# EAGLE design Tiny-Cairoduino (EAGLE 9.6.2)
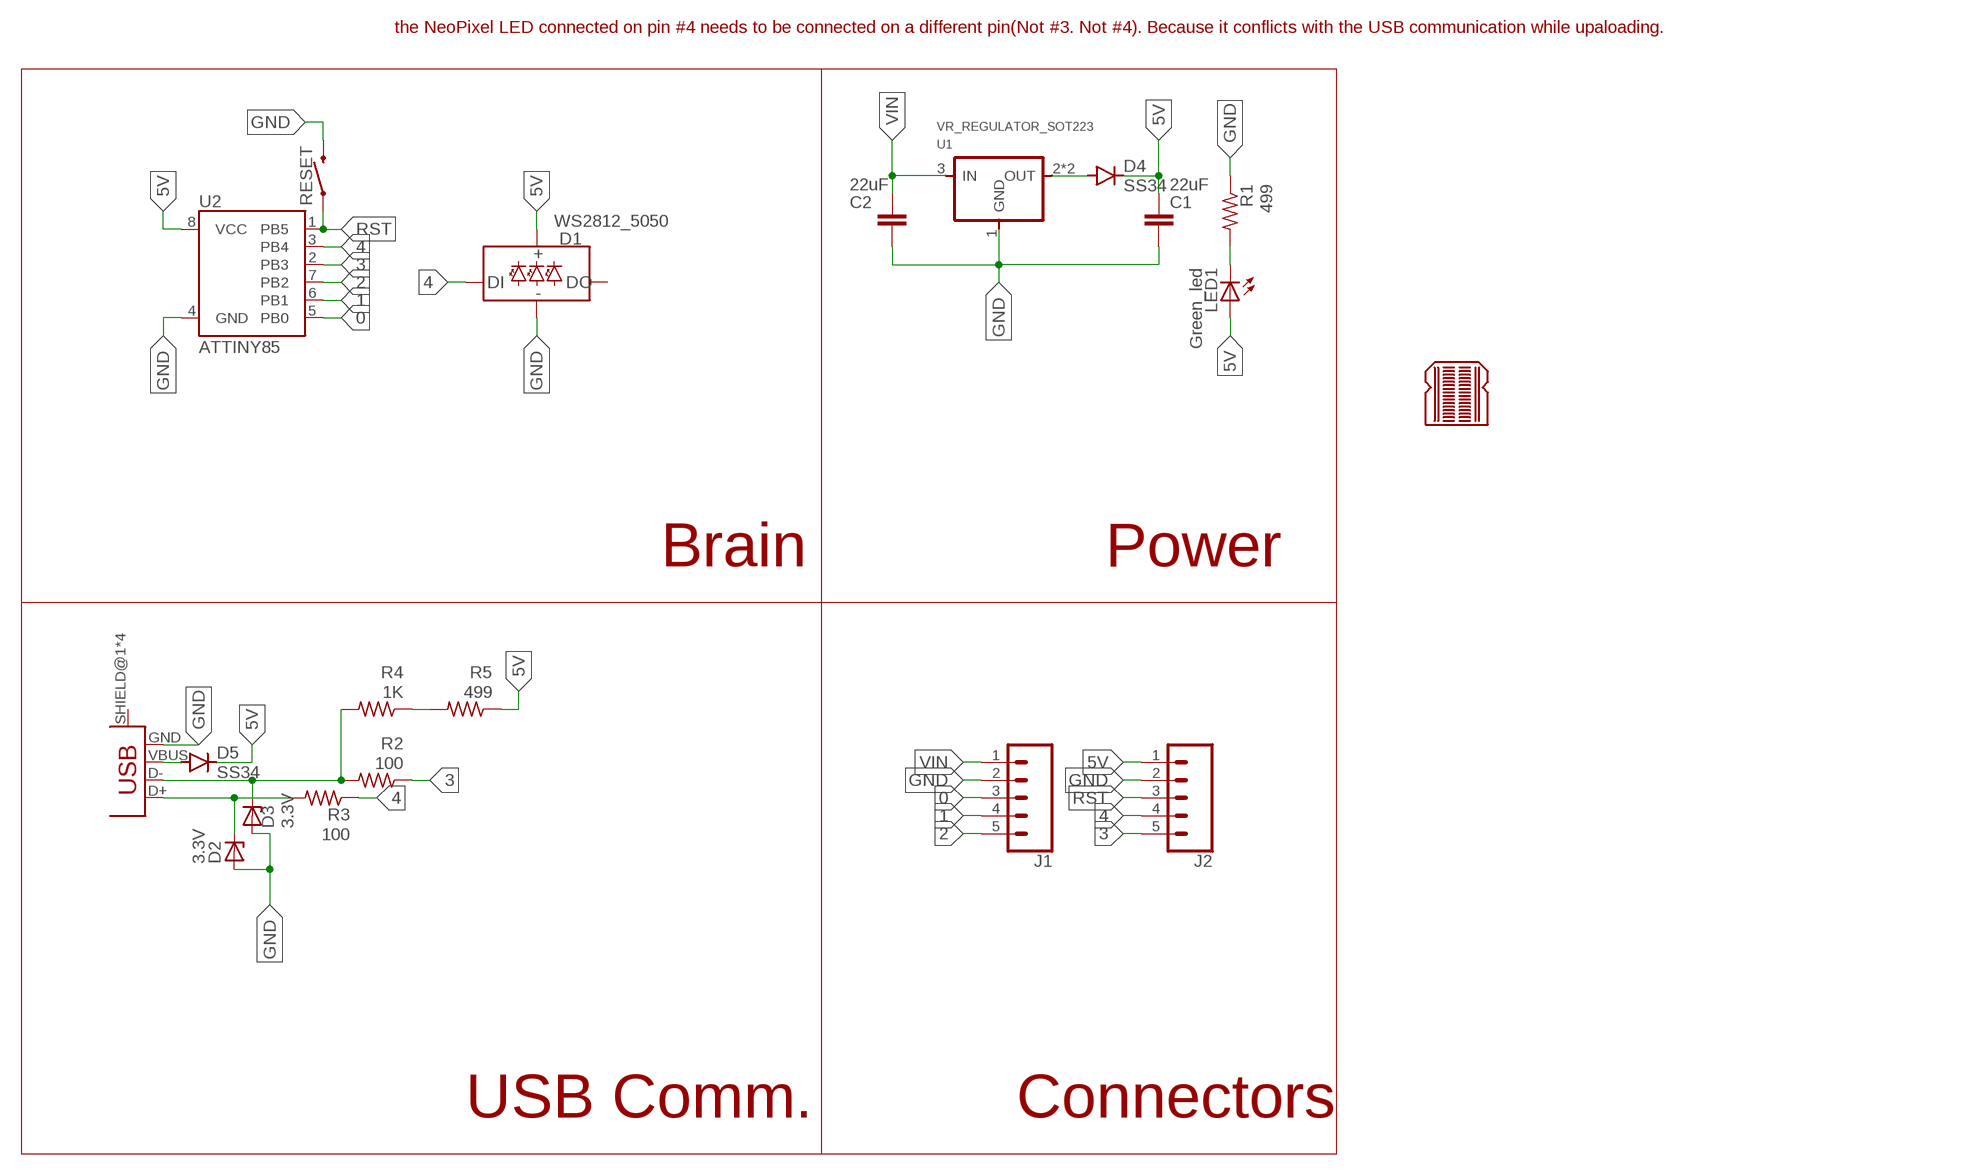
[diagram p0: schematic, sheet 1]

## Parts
C1  22uF  22UF-0805-16V-20%  [0805]
C2  22uF  22UF-0805-16V-20%  [0805]
D1  WS2812_5050  [WS2812-5X5-4PIN]
D2  3.3V  DIODE_ZENERSOD123  [SOD123]
D3  3.3V  DIODE_ZENERSOD123  [SOD123]
D4  SS34  DIODE-DO-214AC  [DO-214AC]
D5  SS34  DIODE-DO-214AC  [DO-214AC]
J1  CONN_05  [1X05]
J2  CONN_05  [1X05]
LED1  Green_led  LEDCHIP-LED0805  [CHIP-LED0805]
LOGO1  BREADBOARD_PATTERN  [BREADBOARD_SPACING]
R1  499  R1206FAB  [R1206FAB]
R2  100  R1206FAB  [R1206FAB]
R3  100  R1206FAB  [R1206FAB]
R4  1K  R1206FAB  [R1206FAB]
R5  499  R1206FAB  [R1206FAB]
RESET  MOMENTARY-SWITCH-SPST-SMD-6.0X3.5MM  [TACTILE_SWITCH_SMD_6.0X3.5MM]
U1  VR_REGULATOR_SOT223  [SOT223]
U2  ATTINY85  [ATTINY85]
U$2  CONN_USB_MINIB  [USB_MINIB]

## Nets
0: J1.3 U2.5(PB0)
1: J1.4 U2.6(PB1)
2: J1.5 U2.7(PB2)
3: J2.5 R2.1 U2.2(PB3)
4: D1.DI J2.4 R3.1 U2.3(PB4)
5V: C1.1 D1.VCC D4.C D5.C J2.1 LED1.A R5.1 U2.8(VCC)
GND: C1.2 C2.2 D1.GND D2.ANODE D3.ANODE J1.2 J2.2 R1.1 RESET.2 U1.1(GND) U2.4(GND) U$2.GND
N$1: LED1.C R1.2
N$2: D5.A U$2.VBUS
N$3: R4.1 R5.2
N$4: D3.CATHODE R2.2 R4.2 U$2.D-
N$5: D2.CATHODE R3.2 U$2.D+
N$6: D4.A U1.2(OUT) U1.4(OUT)
RST: J2.3 RESET.1 U2.1(PB5)
VIN: C2.1 J1.1 U1.3(IN)
Unconnected: D1.DO U$2.SHIELD@1(SHIELD) U$2.SHIELD@2(SHIELD) U$2.SHIELD@3(SHIELD) U$2.SHIELD@4(SHIELD)

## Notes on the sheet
- the NeoPixel LED connected on pin #4 needs to be connected on a different pin(Not #3. Not #4). Because it conflicts with the USB communication while upaloading.
- Brain | Power
- USB Comm. | Connectors

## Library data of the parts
C1 C2 = SparkFun-Capacitors:22UF: 22µF ceramic capacitors; PROD_ID: CAP-14260
D1 = SparkFun-LED:WS2812: Addressable RGB LED - 1 Wire Common names: WS2812, SK6812, Neopixel, APA-106, etc. SMD LED with built-in controller IC. Color: Red/Green/Blue SparkFun Products: LED-SMD RGB (WS2812) LED - RGB Addressable, PTH, 5mm Diffused (5 Pack) LED - RGB Addressable, PTH, 5mm Clear (5 Pack) Blynk Board -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; PROD_ID: DIO-12503
D2 D3 = fab:DIODE_ZENER: zener diode
D4 D5 = diode:DIODE-: DIODE
J1 J2 = SparkFun-Connectors:CONN_05: Multi connection point. Often used as Generic Header-pin footprint for 0.1 inch spaced/style header connections On any of the 0.1 inch spaced packages, you can populate with these: Break Away Headers - Straight (PRT-00116) Break Away Male Headers - Right Angle (PRT-00553) Female Headers (PRT-00115)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
LED1 = adafruit:LED: LED
LOGO1 = SparkFun-Aesthetics:BREADBOARD_PATTERN: Breadboard-Spacing Reference
R1-R5 = fab:R: Resistor (US Symbol)
RESET = SparkFun-Switches:MOMENTARY-SWITCH-SPST: Momentary Switch (Pushbutton) - SPST; PROD_ID: SWCH-14278; SF_SKU: COM-08229
U1 = fab:VR_REGULATOR_SOT223
U2 = SparkFun-IC-Microcontroller:ATTINY85; PROD_ID: IC-09092
U$2 = fab:CONN_USB_MINIB

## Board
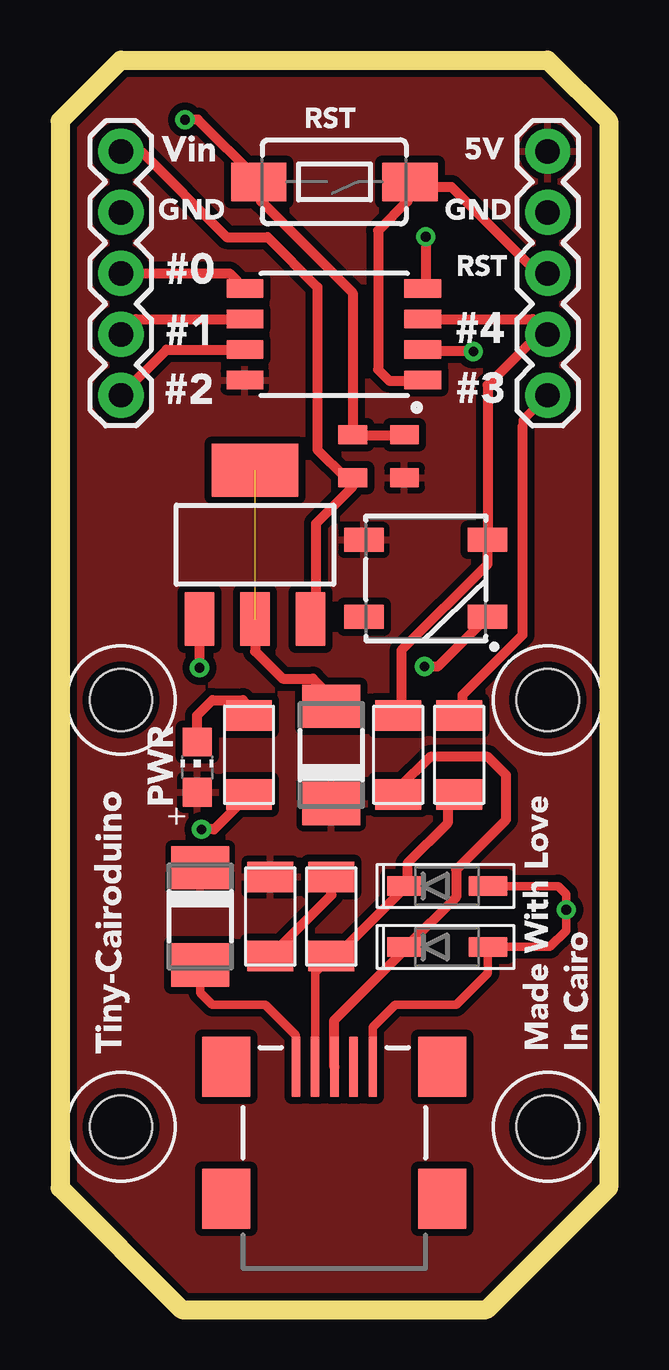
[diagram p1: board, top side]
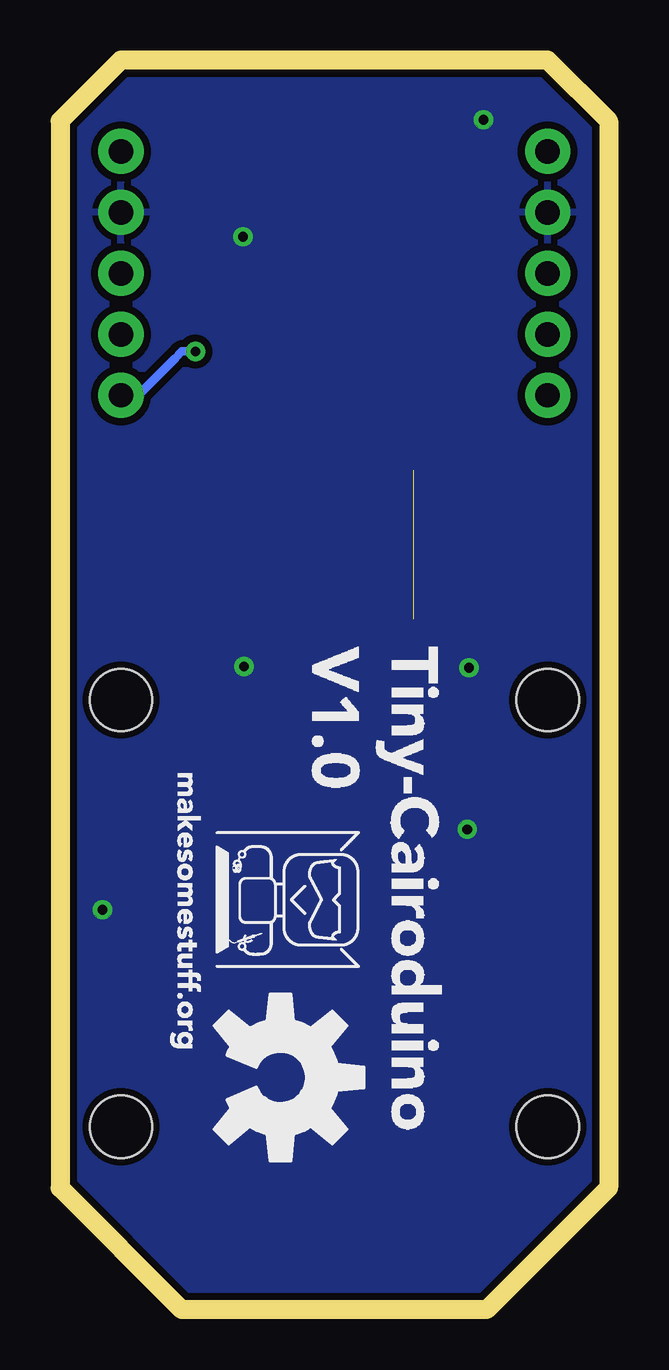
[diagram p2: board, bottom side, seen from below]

Size 22.86 x 52.07 mm. Coordinates in mm from the lower left corner, seen from the top.
Outline: 0,49.53 2.54,52.07 20.32,52.07 22.86,49.53 22.86,5.08 17.78,0 5.08,0 0,5.08 0,49.53
Copper layers (1*16): Top 0.035mm / dielectric 1.5mm / Bottom 0.035mm
Design rules "default *": minimum track width 0.3mm, minimum drill 0.3mm, track to track 10mil, track to pad 10mil, pad to pad 10mil, via to via 10mil, smd to smd 10mil, copper to edge 10mil, drill to drill 10mil, minimum pad ring 10mil, minimum via ring 8mil, stop-mask expansion 4mil, vias tented up to drill 0mil, thermal gap 10mil
Holes 2.6 mm at 20.32,7.62 2.54,7.62 20.32,25.4 2.54,25.4

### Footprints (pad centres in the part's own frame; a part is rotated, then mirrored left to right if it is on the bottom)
0805 = smd 0.8 x 1.2: 1 -0.9,0; 2 0.9,0
WS2812-5X5-4PIN = smd 1.651 x 1: DI 2.577,1.6; DO -2.577,-1.6; GND 2.577,-1.6; VCC -2.577,1.6
SOD123 = smd 1.6 x 0.8: ANODE 1.7,0; CATHODE -1.7,0
DO-214AC = smd 1.8 x 2.4: A 2.025,0; C -2.025,0
1X05 = drill 1.016 pad 1.88: 1 0,0; 2 2.54,0; 3 5.08,0; 4 7.62,0; 5 10.16,0
CHIP-LED0805 = smd 1.2 x 1.2: A 0,-1.05; C 0,1.05
R1206FAB = smd 1.27 x 1.905: 1 -1.651,0; 2 1.651,0
TACTILE_SWITCH_SMD_6.0X3.5MM = smd 2.3 x 1.6: 1 -3.15,0; 2 3.15,0
SOT223 = smd 1.219 x 2.235: 1 -2.311,-3.099; 2 0,-3.099; 3 2.311,-3.099 | smd 3.6 x 2.2: 4 0,3.099
ATTINY85 = smd 1.524 x 0.762: 1 -3.683,1.905; 2 -3.683,0.635; 3 -3.683,-0.635; 4 -3.683,-1.905; 5 3.727,-1.905; 6 3.727,-0.635; 7 3.727,0.635; 8 3.727,1.905
USB_MINIB = smd 2.5 x 0.35: D+ 3.77,0; D- 3.77,0.8; GND 3.77,-1.6; ID 3.77,-0.8; VBUS 3.77,1.6 | smd 2.5 x 2: SHIELD@1 -1.73,-4.5; SHIELD@2 -1.73,4.5; SHIELD@3 3.77,4.5; SHIELD@4 3.77,-4.5

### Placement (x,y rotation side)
C1  14.35,35.56 90 top
C2  12.19,35.56 90 top
D1  15.24,30.48 0 top
D2  16.13,15.11 0 top
D3  16.13,17.65 0 top
D4  11.3,23.11 90 top
D5  5.84,16.38 270 top
J1  2.54,48.26 270 top
J2  20.32,48.26 270 top
LED1  5.71,22.61 0 top
LOGO1  not placed on the board
R1  7.87,23.11 90 top
R2  16.64,23.11 270 top
R3  14.1,23.11 270 top
R4  11.3,16.38 270 top
R5  8.76,16.38 270 top
RESET  11.43,46.99 180 top
U1  8.13,31.88 0 top
U2  11.43,40.64 180 top
U$1  [OSHW-LOGO-L]  13.68,9.68 270 bottom
U$2  11.43,6.35 90 top

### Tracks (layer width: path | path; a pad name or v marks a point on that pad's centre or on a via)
0
  Top 0.406: J1.3 7.07,43.18 U2.5
1
  Top 0.406: J1.4 3.17,41.27 U2.6
2
  Top 0.406: J1.5 4.45,40.01 U2.7
3  (via drill 0.4)
  Top 0.35: 19.28,36.8 19.28,37.06 J2.5
  Top 0.406: v17.22,39.93 15.24,39.93 U2.2 | R2.1 16.76,24.84 16.76,25.6 19.28,28.12 19.28,36.8
  Bottom 0.35: J2.5 19.61,38.1 18.06,39.65 17.78,39.93 v17.22,39.93
4
  Top 0.406: R3.1 14.22,24.89 14.22,27.47 17.82,31.06 D1.DI 17.82,38.52 19.94,40.64 J2.4 19.68,41.27 U2.3
5V
  pour Top (isolate 0.3): 5.08,0 0,5.08 0,49.53 2.54,52.07 20.32,52.07 22.86,49.53 22.86,5.08 17.78,0
GND  (via drill 0.4)
  Top 0.35: U$2.GND 13.03,11.76 13.97,12.7 16.51,12.7 17.83,14.02 D2.ANODE 20.41,15.11 21.09,15.8 v21.09,16.66 21.09,17.31 20.75,17.65 D3.ANODE
  Top 0.406: 17.83,17.53 D3.ANODE | C1.2 14.33,36.42 12.19,36.42 C2.2 12.19,42.37 8.38,46.18 8.38,46.94 RESET.2 8.23,47.09 5.74,49.58 v5.21,49.58 | v15.24,44.7 15.24,42.67 U2.4 | D1.GND 15.73,26.8 v15.19,26.8 | R1.1 6.43,20.02 v5.89,20.02 | v5.82,26.75 U1.1
  pour Bottom (isolate 0.3): 5.08,0 0,5.08 0,49.53 2.54,52.07 20.32,52.07 22.86,49.53 22.86,5.08 17.78,0
N$1
  Top 0.406: LED1.C 5.71,24.77 6.35,25.4 7.62,25.4 7.87,25.15 R1.2
N$2
  Top 0.35: D5.A 5.84,13.21 6.35,12.7 8.56,12.7 9.83,11.43 U$2.VBUS
N$3
  Top 0.406: R5.2 11.3,17.27 R4.1
N$4
  Top 0.35: U$2.D- 10.63,14.06 R4.2
  Top 0.406: R2.2 16.61,21.34 16.15,20.88 16.15,20.27 14.48,18.59 14.48,17.68 D3.CATHODE 11.51,14.73 R4.2
N$5
  Top 0.406: R3.2 14.1,21.72 15.42,23.04 17.83,23.04 18.59,22.28 18.59,20.42 16.51,18.34 16.51,17.19 D2.CATHODE 14.43,15.06 11.43,12.06 U$2.D+
N$6  (1 unrouted)
  Top 0.406: U1.2 8.13,27.43 9.27,26.29 10.54,26.29 11.3,25.53 D4.A
RST
  Top 0.406: 14.48,46.79 14.48,46.94 RESET.1 14.48,46.79 | 14.48,46.79 14.48,46.18 13.26,44.96 13.26,39.17 13.72,38.71 15.09,38.71 U2.1 | 14.48,46.79 16.31,46.79 19.81,43.28 20.27,43.28 J2.3
VIN
  Top 0.406: U1.3 10.52,28.8 10.67,28.96 10.67,32.77 12.19,34.29 C2.1 11.91,34.66 10.73,35.84 10.73,42.61 8.65,44.69 6.95,44.69 3.38,48.26 J1.1

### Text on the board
Measures: the NeoPixel LED connected on pin #4 needs to be connected on a different pin(Not #3. Not #4). Because it conflicts with the USB communication while uploading.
